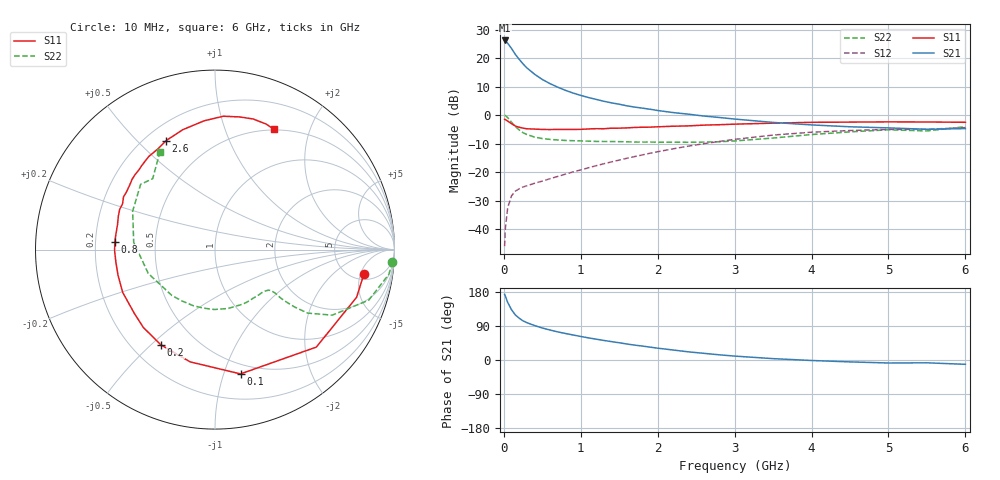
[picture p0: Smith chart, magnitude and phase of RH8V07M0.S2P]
! SIEMENS Small Signal Semiconductors
! BFR106
! Si NPN RF Bipolar Junction Transistor in SOT23
! VCE = 8 V  IC = 7 mA
! Common Emitter S-Parameters:  August  1996
# GHz  S  MA  R  50
!  f  S11  S21  S12  S22
! GHz  MAG  ANG  MAG  ANG  MAG  ANG  MAG  ANG
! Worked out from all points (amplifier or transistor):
!   36 points, 10 MHz to 6 GHz, reference 50 ohm
!   highest |S21| = 26.2 dB at 10 MHz (marker M1)
!   |S21| within 3 dB of that: start of sweep to 104.2 MHz
!   unconditionally stable (mu >= 1): 558.8 MHz to 1.917 GHz; 5.165 GHz to end of sweep
!   at 250 MHz: K = 0.59, MSG = 21.6 dB, |S12| = -25.3 dB
!   at 1.4 GHz: K = 1.11, MAG = 8.4 dB, |S12| = -16.4 dB
!   at 6 GHz: K = 1.01, MAG = -0.9 dB, |S12| = -4.4 dB
!   S11 on the Smith chart (normalised r, x): 10 MHz: 6.05, -5.71; 100 MHz: 0.41, -1.14; 200 MHz: 0.32, -0.54; 800 MHz: 0.28, +0.03; 2.6 GHz: 0.28, +0.61; 6 GHz: 0.49, +1.49
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0.01  0.8403 -9.5  20.35 173.2  0.005 86.9  0.991 -4.0
0.02  0.8325 -18.6  20.04 168.2  0.0103 79.0  0.9784 -8.1
0.05  0.7834 -43.9  18.16 151.9  0.0236 68.5  0.9017 -18.2
0.1  0.707 -78.4  14.7 132.7  0.0383 55.5  0.7486 -29.2
0.15  0.6407 -102.5  11.57 118.8  0.0463 47.1  0.6263 -34.4
0.2  0.6104 -119.7  9.482 110.2  0.0508 44.4  0.5476 -35.8
0.25  0.5896 -132.6  7.879 103.2  0.0546 43.3  0.4888 -36.3
0.3  0.5732 -141.5  6.71 98.5  0.0575 44.3  0.4548 -36.4
0.4  0.5669 -155.1  5.195 90.9  0.0635 46.2  0.4103 -35.9
0.5  0.5589 -165.2  4.206 84.4  0.0693 49.2  0.3865 -36.1
0.6  0.5566 -172.7  3.556 79.1  0.0763 51.7  0.3738 -37.2
0.8  0.5598 175.8  2.714 70.0  0.0917 56.4  0.3579 -40.8
1.1  0.5698 160.9  2.029 58.4  0.1187 61.3  0.3482 -48.5
1.3  0.5747 153.6  1.744 51.6  0.1398 63.0  0.3433 -54.6
1.6  0.5948 143.4  1.45 42.2  0.1743 63.7  0.339 -65.3
2.2  0.6365 125.5  1.105 26.4  0.2552 60.5  0.3338 -90.7
2.6  0.6654 114.2  0.96 17.6  0.3142 55.5  0.3351 -111.2
3.5  0.7203 94.8  0.742 3.6  0.4448 40.5  0.3947 -160.3
4.5  0.7519 79.4  0.622 -5.0  0.5352 21.4  0.5063 155.0
5  0.7582 73.7  0.595 -7.9  0.5597 13.2  0.5513 138.7
5.5  0.7552 67.8  0.562 -7.4  0.5616 8.7  0.526 131.3
6  0.7465 64.0  0.578 -11.4  0.6015 0.6  0.6248 119.4
